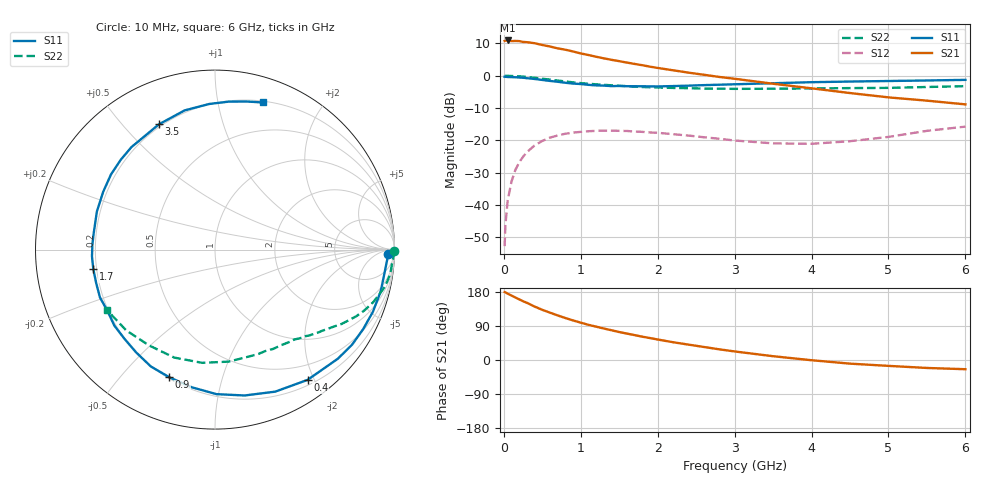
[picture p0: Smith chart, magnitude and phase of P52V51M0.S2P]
! SIEMENS Small Signal Semiconductors
! BFP183
! Si NPN RF Bipolar Junction Transistor in SOT143
! VCE = 2.5 V  IC = 1 mA
! Common Emitter S-Parameters:  March  1996
# GHz  S  MA  R  50
!  f  S11  S21  S12  S22
! GHz  MAG  ANG  MAG  ANG  MAG  ANG  MAG  ANG
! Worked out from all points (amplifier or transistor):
!   36 points, 10 MHz to 6 GHz, reference 50 ohm
!   highest |S21| = 10.9 dB at 50 MHz (marker M1)
!   |S21| within 3 dB of that: start of sweep to 824.7 MHz
!   unconditionally stable (mu >= 1): 2.473 GHz to end of sweep
!   at 250 MHz: K = 0.10, MSG = 17.8 dB, |S12| = -25.1 dB
!   at 1.4 GHz: K = 0.55, MSG = 11.0 dB, |S12| = -17.0 dB
!   at 6 GHz: K = 1.05, MAG = 2.1 dB, |S12| = -15.8 dB
!   S11 on the Smith chart (normalised r, x): 10 MHz: 37, -24; 400 MHz: 0.27, -1.91; 900 MHz: 0.21, -0.68; 1.7 GHz: 0.19, -0.08; 3.5 GHz: 0.19, +0.63; 6 GHz: 0.21, +1.35
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0.01  0.9633 -1.4  3.456 179.3  0.0023 87.3  0.9999 -0.5
0.02  0.9619 -3.0  3.485 178.6  0.0048 85.1  0.9969 -1.0
0.05  0.9541 -7.3  3.512 175.0  0.0118 87.3  0.9947 -2.5
0.1  0.9521 -14.1  3.432 170.1  0.0231 81.8  0.9884 -5.0
0.15  0.9456 -21.5  3.45 164.9  0.0349 76.6  0.9863 -7.5
0.2  0.937 -28.2  3.433 160.0  0.0457 73.2  0.9784 -9.8
0.25  0.9294 -34.8  3.332 155.1  0.0556 69.0  0.9697 -12.2
0.3  0.9155 -41.6  3.304 150.9  0.0658 64.9  0.9548 -14.3
0.4  0.8904 -54.6  3.183 141.0  0.0831 57.5  0.9288 -18.4
0.5  0.8597 -67.0  2.986 132.4  0.0979 50.1  0.8982 -22.2
0.6  0.8294 -78.5  2.832 124.9  0.1101 43.9  0.8699 -25.3
0.8  0.778 -99.5  2.525 110.7  0.1265 33.2  0.8161 -30.6
0.9  0.7553 -109.7  2.372 104.4  0.1317 28.4  0.7893 -32.9
1.1  0.7218 -127.5  2.091 92.8  0.1383 20.3  0.7502 -37.0
1.4  0.6896 -150.2  1.761 78.5  0.141 10.4  0.7106 -42.3
1.7  0.6866 -170.8  1.522 65.7  0.1368 3.5  0.6761 -47.3
2.2  0.6915 162.1  1.213 46.9  0.1245 -4.4  0.6466 -55.7
2.8  0.7253 136.5  0.957 28.2  0.1058 -7.2  0.6296 -67.3
3.5  0.7648 114.1  0.751 10.0  0.0897 0.2  0.6288 -83.1
4.5  0.812 92.3  0.539 -9.6  0.0968 19.0  0.6431 -110.7
5.5  0.8437 77.9  0.411 -21.0  0.1402 25.9  0.6688 -137.7
6  0.8619 72.0  0.36 -24.3  0.1629 23.1  0.6888 -150.5
